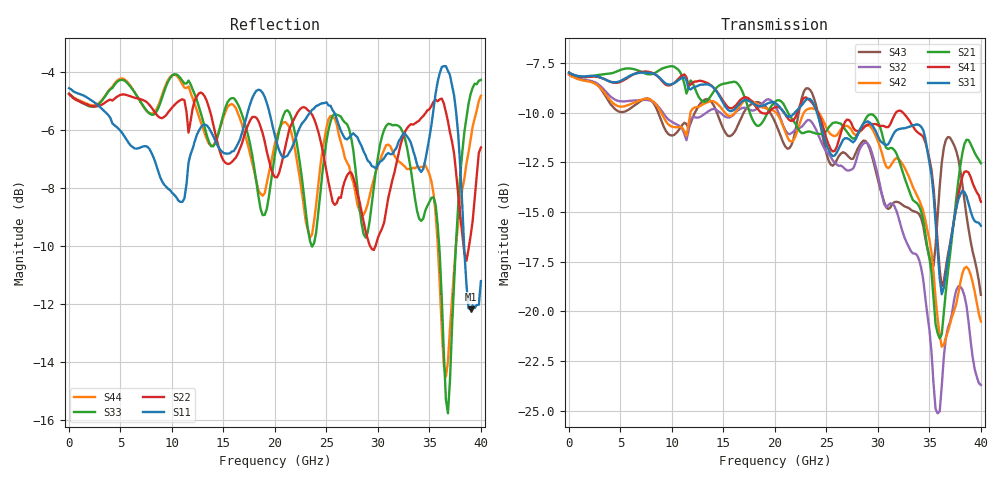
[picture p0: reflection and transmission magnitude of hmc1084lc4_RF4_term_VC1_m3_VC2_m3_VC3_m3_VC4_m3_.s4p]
!Agilent Technologies,N5224A,MY51441122,A.09.40.06
!Agilent N5224A: A.09.40.06
!Date: Thursday, June 19, 2014 00:53:19
!Correction: S11(Full 4 Port(1,2,3,4))
!S12(Full 4 Port(1,2,3,4))
!S13(Full 4 Port(1,2,3,4))
!S14(Full 4 Port(1,2,3,4))
!S21(Full 4 Port(1,2,3,4))
!S22(Full 4 Port(1,2,3,4))
!S23(Full 4 Port(1,2,3,4))
!S24(Full 4 Port(1,2,3,4))
!S31(Full 4 Port(1,2,3,4))
!S32(Full 4 Port(1,2,3,4))
!S33(Full 4 Port(1,2,3,4))
!S34(Full 4 Port(1,2,3,4))
!S41(Full 4 Port(1,2,3,4))
!S42(Full 4 Port(1,2,3,4))
!S43(Full 4 Port(1,2,3,4))
!S44(Full 4 Port(1,2,3,4))
!S4P File: Measurements: <S11,S12,S13,S14>,
!<S21,S22,S23,S24>,
!<S31,S32,S33,S34>,
!<S41,S42,S43,S44>:
# Hz S  dB  R 50
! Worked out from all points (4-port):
!   201 points, 10 MHz to 40 GHz, reference 50 ohm
!   strongest paths, dB at 10 MHz, 10.01 GHz, 20 GHz, 30 GHz, 40 GHz:
!     S31: -8.0, -8.6, -9.5, -11.2, -15.7
!     S41: -8.0, -8.6, -9.7, -10.6, -14.5
!     S21: -8.0, -7.7, -9.5, -10.5, -12.5
!     S42: -8.1, -10.7, -10.0, -11.4, -20.5
!     S32: -8.1, -10.5, -9.6, -13.2, -23.7
!     S43: -8.1, -11.2, -10.5, -13.4, -19.2
!   lowest |S11| = -12.2 dB at 39 GHz (marker M1), VSWR 1.65, Z = 30.5 + j3.4 ohm
!   |S11| at or under -10 dB: 38.37 GHz to end of sweep
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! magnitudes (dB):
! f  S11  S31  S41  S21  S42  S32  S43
! 10 MHz  -4.6  -8.0  -8.0  -8.0  -8.1  -8.1  -8.1
! 23.6 GHz  -5.3  -9.4  -9.5  -11.0  -9.8  -10.5  -9.0
! 32 GHz  -6.4  -10.8  -9.9  -12.3  -12.3  -15.3  -14.5
! 35.4 GHz  -5.3  -14.1  -13.8  -19.3  -18.0  -23.6  -17.7
! 36.8 GHz  -4.0  -17.3  -17.1  -18.0  -21.0  -20.8  -11.2
! 39 GHz  -12.2  -14.9  -13.2  -11.6  -18.1  -21.5  -16.5
! 40 GHz  -11.2  -15.7  -14.5  -12.5  -20.5  -23.7  -19.2
